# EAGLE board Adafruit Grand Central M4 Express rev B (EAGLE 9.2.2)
REV: B
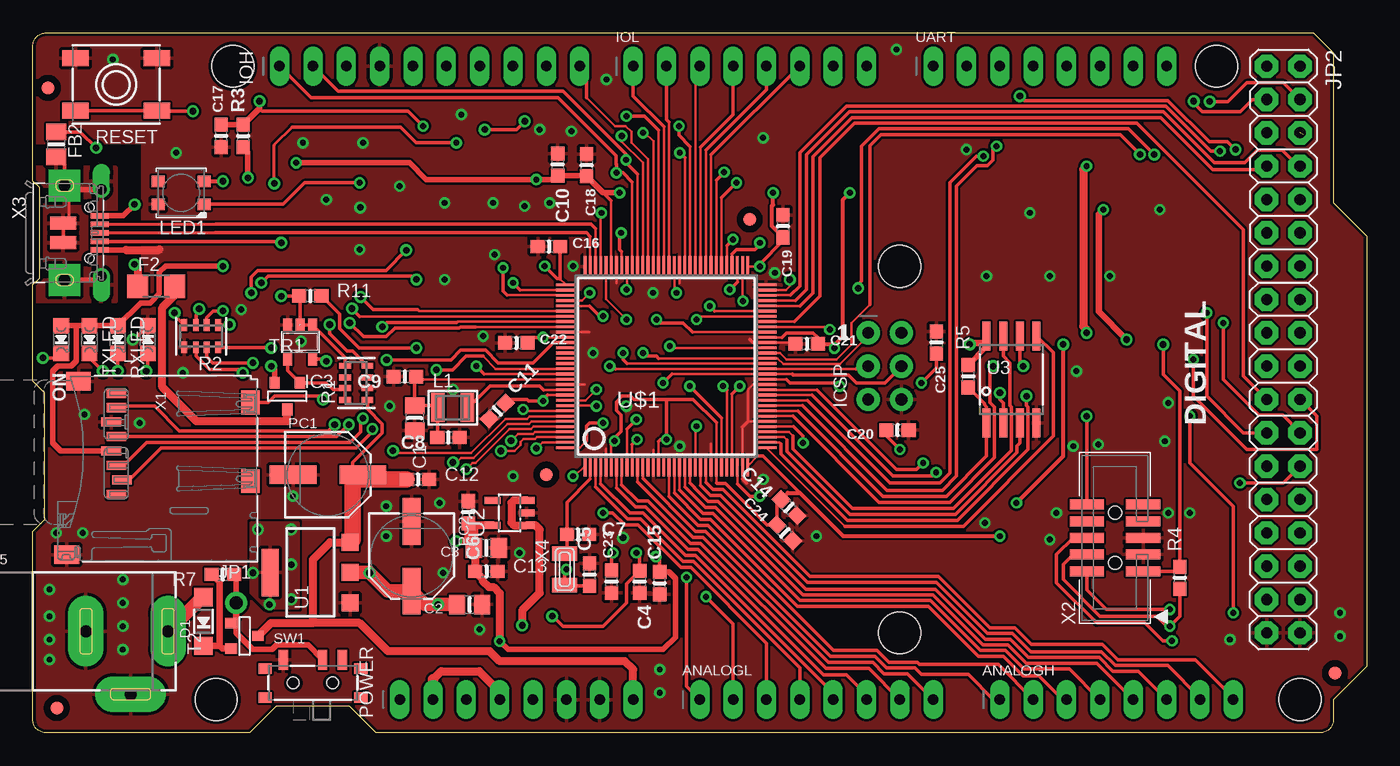
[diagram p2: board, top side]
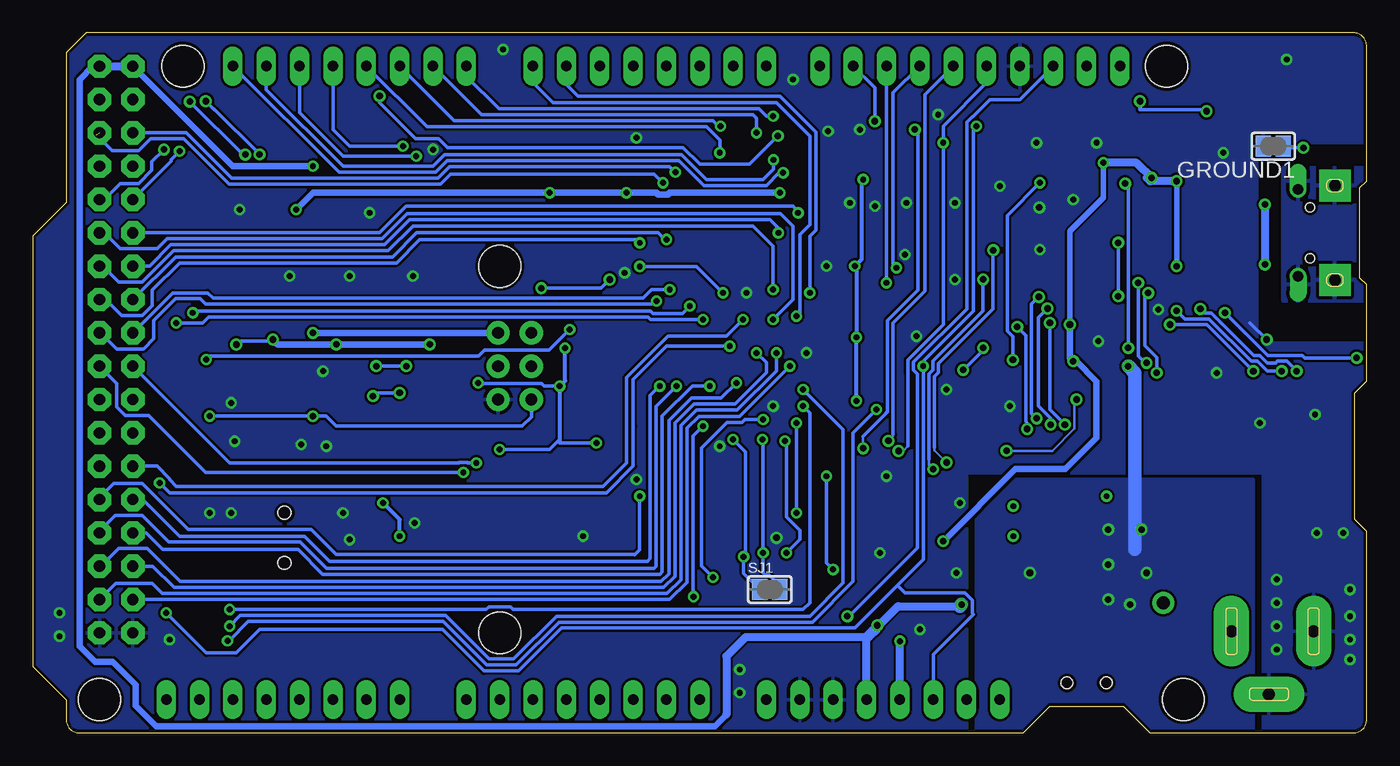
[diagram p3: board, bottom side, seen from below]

Size 101.6 x 53.34 mm. Coordinates in mm from the lower left corner, seen from the top.
Outline: 97.54,53.34 99.06,51.82 99.06,40.39 101.6,37.85 101.6,5.08 99.06,2.54 99.06,1 arc-90 98.06,0 26.16,0 24.13,2.03 18.54,2.03 16.51,0 1,0 arc-90 0,1 0,15.37 0.89,16.26 0.89,25.91 0,26.8 0,34.16 0.51,34.67 0.51,41.53 0,42.04 0,52.34 arc-90 1,53.34 97.54,53.34
Copper layers (1*16): Top 0.035mm / dielectric 1.5mm / Bottom 0.035mm
Design rules "adafruit *": minimum track width 7mil, minimum drill 15.5mil, track to track 7mil, track to pad 7mil, pad to pad 7mil, via to via 7mil, smd to smd 7mil, copper to edge 10mil, drill to drill 8mil, minimum pad ring 10mil, minimum via ring 8mil, stop-mask expansion 2mil, vias tented up to drill 20mil, thermal gap 10mil
Holes 3.2 mm at 66.04,35.56 66.04,7.62 15.24,50.8 13.97,2.54 96.52,2.54 90.17,50.8

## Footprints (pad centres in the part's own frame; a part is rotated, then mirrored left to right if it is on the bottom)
1X08_OVALWAVE = drill 0.8 pad 1.5 long: 1 -8.89,0; 2 -6.35,0; 3 -3.81,0; 4 -1.27,0; 5 1.27,0; 6 3.81,0; 7 6.35,0; 8 8.89,0
0805-NO = smd 1.24 x 1.5: 1 -0.95,0; 2 0.95,0
0603-NO = smd 1.075 x 1: 1 -0.85,0; 2 0.85,0
SOD-123 = smd 1.4 x 1.4: A 1.85,0; C -1.85,0
R1206 = smd 1.6 x 1.803: 1 -1.422,0; 2 1.422,0
FIDUCIAL_1MM = smd 1 x 1: 1 0,0
SOLDERJUMPER_CLOSEDWIRE = smd 1.168 x 1.6: 1 -0.762,0; 2 0.762,0 | smd 0.635 x 0.203: WIRE 0,0
SOT23-5 = smd 0.69 x 0.99: 1 -0.95,-1.29; 2 0,-1.29; 3 0.95,-1.29; 4 0.95,1.3; 5 -0.95,1.3
2X03_ROUND_70MIL = drill 0.9 pad 1.778: 1 -2.54,-1.27; 2 -2.54,1.27; 3 0,-1.27; 4 0,1.27; 5 2.54,-1.27; 6 2.54,1.27
1X10_OVALWAVE = drill 0.8 pad 1.5 long: 1 -11.43,0; 2 -8.89,0; 3 -6.35,0; 4 -3.81,0; 5 -1.27,0; 6 1.27,0; 7 3.81,0; 8 6.35,0; 9 8.89,0; 10 11.43,0
1X01_ROUND = drill 1 pad 1.676: 1 0,0
2X18_THICKWAVE = drill 0.85 pad 1.778 octagon: 1 -21.59,-1.27; 2 -21.59,1.27; 3 -19.05,-1.27; 4 -19.05,1.27; 5 -16.51,-1.27; 6 -16.51,1.27; 7 -13.97,-1.27; 8 -13.97,1.27; 9 -11.43,-1.27; 10 -11.43,1.27; 11 -8.89,-1.27; 12 -8.89,1.27; 13 -6.35,-1.27; 14 -6.35,1.27; 15 -3.81,-1.27; 16 -3.81,1.27; 17 -1.27,-1.27; 18 -1.27,1.27; 19 1.27,-1.27; 20 1.27,1.27; 21 3.81,-1.27; 22 3.81,1.27; 23 6.35,-1.27; 24 6.35,1.27; 25 8.89,-1.27; 26 8.89,1.27; 27 11.43,-1.27; 28 11.43,1.27; 29 13.97,-1.27; 30 13.97,1.27; 31 16.51,-1.27; 32 16.51,1.27; 33 19.05,-1.27; 34 19.05,1.27; 35 21.59,-1.27; 36 21.59,1.27
CHIPLED_0805_NOOUTLINE = smd 1.2 x 1.2: A 0,-1.05; C 0,1.05
INDUCTOR_1007 = smd 1.016 x 2.2: P$1 -1.127,0; P$2 1.127,0
LED3535 = smd 1 x 0.85: 1 -1.75,0.875; 2 -1.75,-0.875; 3 1.75,-0.875; 4 1.75,0.875
PANASONIC_D = smd 3.556 x 1.4: + 2.654,0; - -2.654,0
RESPACK_4X0603 = smd 0.45 x 0.9: 1 -1.3,-0.85; 2 -0.4,-0.85; 3 0.4,-0.85; 4 1.3,-0.85; 5 1.3,0.85; 6 0.4,0.85; 7 -0.4,0.85; 8 -1.3,0.85
EVQ-Q2_SMALLER = smd 2 x 1.2: A -3.1,-2; A' 3.1,-2; B -3.1,2; B' 3.1,2
SPDT_SMT_SSSS811101 = smd 0.7 x 1.5: A -2.25,1.75; B 0.75,1.75; C 2.25,1.75 | smd 1 x 0.8: SUP1 -3.65,1.1; SUP2 -3.65,-1.1; SUP3 3.65,1.1; SUP4 3.65,-1.1 | hole 0.9: -1.5,0; 1.5,0
SOT-23 = smd 0.787 x 0.889: 1 0.025,-1.016; 2 -0.94,1.016; 3 0.991,1.016
SOT223-R = smd 1.3 x 1.3: 1 -2.3,-3.05; 2 0,-3.05; 3 2.3,-3.05 | smd 3.6 x 1.3: 4 0,3.05
SOT23-DBV = smd 0.55 x 1.2: 1 -0.95,-1.3; 2 0,-1.3; 3 0.95,-1.3; 4 0.95,1.3; 5 -0.95,1.3
SOIC8_208MIL = smd 0.6 x 2.2: 1 -1.905,-3.315; 2 -0.635,-3.315; 3 0.635,-3.315; 4 1.905,-3.315; 5 1.905,3.315; 6 0.635,3.315; 7 -0.635,3.315; 8 -1.905,3.315
SQFP-S-14X14-128 = smd 0.2 x 1.6: 1 -6.2,-7.6; 2 -5.8,-7.6; 3 -5.4,-7.6; 4 -5,-7.6; 5 -4.6,-7.6; 6 -4.2,-7.6; 7 -3.8,-7.6; 8 -3.4,-7.6; 9 -3,-7.6; 10 -2.6,-7.6; 11 -2.2,-7.6; 12 -1.8,-7.6; 13 -1.4,-7.6; 14 -1,-7.6; 15 -0.6,-7.6; 16 -0.2,-7.6; 17 0.2,-7.6; 18 0.6,-7.6; 19 1,-7.6; 20 1.4,-7.6; 21 1.8,-7.6; 22 2.2,-7.6; 23 2.6,-7.6; 24 3,-7.6; 25 3.4,-7.6; 26 3.8,-7.6; 27 4.2,-7.6; 28 4.6,-7.6; 29 5,-7.6; 30 5.4,-7.6; 31 5.8,-7.6; 32 6.2,-7.6; 65 6.2,7.6; 66 5.8,7.6; 67 5.4,7.6; 68 5,7.6; 69 4.6,7.6; 70 4.2,7.6; 71 3.8,7.6; 72 3.4,7.6; 73 3,7.6; 74 2.6,7.6; 75 2.2,7.6; 76 1.8,7.6; 77 1.4,7.6; 78 1,7.6; 79 0.6,7.6; 80 0.2,7.6; 81 -0.2,7.6; 82 -0.6,7.6; 83 -1,7.6; 84 -1.4,7.6; 85 -1.8,7.6; 86 -2.2,7.6; 87 -2.6,7.6; 88 -3,7.6; 89 -3.4,7.6; 90 -3.8,7.6; 91 -4.2,7.6; 92 -4.6,7.6; 93 -5,7.6; 94 -5.4,7.6; 95 -5.8,7.6; 96 -6.2,7.6 | smd 1.6 x 0.2: 33 7.6,-6.2; 34 7.6,-5.8; 35 7.6,-5.4; 36 7.6,-5; 37 7.6,-4.6; 38 7.6,-4.2; 39 7.6,-3.8; 40 7.6,-3.4; 41 7.6,-3; 42 7.6,-2.6; 43 7.6,-2.2; 44 7.6,-1.8; 45 7.6,-1.4; 46 7.6,-1; 47 7.6,-0.6; 48 7.6,-0.2; 49 7.6,0.2; 50 7.6,0.6; 51 7.6,1; 52 7.6,1.4; 53 7.6,1.8; 54 7.6,2.2; 55 7.6,2.6; 56 7.6,3; 57 7.6,3.4; 58 7.6,3.8; 59 7.6,4.2; 60 7.6,4.6; 61 7.6,5; 62 7.6,5.4; 63 7.6,5.8; 64 7.6,6.2; 97 -7.6,6.2; 98 -7.6,5.8; 99 -7.6,5.4; 100 -7.6,5; 101 -7.6,4.6; 102 -7.6,4.2; 103 -7.6,3.8; 104 -7.6,3.4; 105 -7.6,3; 106 -7.6,2.6; 107 -7.6,2.2; 108 -7.6,1.8; 109 -7.6,1.4; 110 -7.6,1; 111 -7.6,0.6; 112 -7.6,0.2; 113 -7.6,-0.2; 114 -7.6,-0.6; 115 -7.6,-1; 116 -7.6,-1.4; 117 -7.6,-1.8; 118 -7.6,-2.2; 119 -7.6,-2.6; 120 -7.6,-3; 121 -7.6,-3.4; 122 -7.6,-3.8; 123 -7.6,-4.2; 124 -7.6,-4.6; 125 -7.6,-5; 126 -7.6,-5.4; 127 -7.6,-5.8; 128 -7.6,-6.2
MICROSD = smd 0.7 x 1.5: 1 9,-10.64; 2 7.9,-10.24; 3 6.8,-10.64; 4 5.7,-11.04; 5 4.6,-10.64; 6 3.5,-11.04; 7 2.4,-10.64; 8 1.3,-10.64 | smd 1.8 x 1.4: CD1 2,-0.44; CD2 8,-0.44 | smd 1.4 x 1.9: MT1 0.4,-13.54; MT2 13.6,-14.44
2X05_1.27MM_BOX_POSTS = smd 0.76 x 2.6: 1 -2.54,-2.15; 2 -2.54,2.15; 3 -1.27,-2.15; 4 -1.27,2.15; 5 0,-2.15; 6 0,2.15; 7 1.27,-2.15; 8 1.27,2.15; 9 2.54,-2.15; 10 2.54,2.15 | hole 1: -1.905,0; 1.905,0
4UCONN_20329_V2 = smd 1 x 2: BASE@1 -0.75,-2; BASE@2 0.75,-2 | smd 0.4 x 1.35: D+ 0,0.775; D- -0.65,0.775; GND 1.3,0.775; ID 0.65,0.775; VBUS -1.3,0.775 | drill 0.8 pad 1.143 offset: SPRT@1 -3.3,0.9; SPRT@2 3.3,0.9 | drill 0.9 pad 2.413 square: SPRT@3 -3.6,-1.9; SPRT@4 3.6,-1.9 | hole 0.7: -1.95,0; 1.95,0
XTAL3215 = smd 1.1 x 1.9: P$1 1.2,0; P$2 -1.2,0
DCJACK_2MM_PTH = drill 0.9 pad 2.7 long: GND 7.35,0; GNDBREAK 10.75,-4.8; PWR 13.6,0

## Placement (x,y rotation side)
ANALOGH  20610  [1X08_OVALWAVE]  82.55,2.54 0 top
ANALOGL  20610  [1X08_OVALWAVE]  59.69,2.54 0 top
C1  10uF  [0805-NO]  29.09,23.98 270 top
C2  10uF  [0805-NO]  33.27,9.78 180 top
C3  10uF  [0805-NO]  34.54,14.1 180 top
C4  .1u  [0603-NO]  46.23,11.51 270 top
C5  22pF  [0603-NO]  42.42,12.06 90 top
C6  .1u  [0603-NO]  33.17,16.8 270 top
C7  22pF  [0603-NO]  41.53,15.11 0 top
C8  .1u  [0603-NO]  31.67,22.5 180 top
C9  1uF  [0603-NO]  28.34,27.14 180 top
C10  .1u  [0603-NO]  39.98,43.3 270 top
C11  .1u  [0603-NO]  35.38,24.53 45 top
C12  0.1uF  [0603-NO]  29.34,19.3 0 top
C13  0.1uF  [0603-NO]  34.54,12.32 0 top
C14  .1u  [0603-NO]  57.6,17.17 135 top
C15  .1u  [0603-NO]  47.75,11.4 90 top
C16  .1u  [0603-NO]  39.32,37.06 0 top
C17  0.1uF  [0603-NO]  14.35,45.49 90 top
C18  .1u  [0603-NO]  42.19,43.26 270 top
C19  .1u  [0603-NO]  57.15,38.61 270 top
C20  .1u  [0603-NO]  65.86,23.06 180 top
C21  .1u  [0603-NO]  58.95,29.64 0 top
C22  .1u  [0603-NO]  36.83,29.72 0 top
C23  .1u  [0603-NO]  44.07,11.53 90 top
C24  .1u  [0603-NO]  57.28,15.24 135 top
C25  .1u  [0603-NO]  68.83,29.74 270 top
D1  MBR120  [SOD-123]  13,8.48 90 top
F2  500mA  [R1206]  9.4,34.04 0 top
FB2  FERRITE  [0805-NO]  1.78,44.83 270 top
FD1  FIDUCIAL_1MM  [FIDUCIAL_1MM]  1.14,49.15 0 top
FD2  FIDUCIAL_1MM  [FIDUCIAL_1MM]  99.18,4.55 0 top
FD3  FIDUCIAL_1MM  [FIDUCIAL_1MM]  1.82,1.89 0 top
FD4  FIDUCIAL_1MM  [FIDUCIAL_1MM]  39.12,19.68 0 top
FD5  FIDUCIAL_1MM  [FIDUCIAL_1MM]  54.61,39.12 0 top
GROUND1  [SOLDERJUMPER_CLOSEDWIRE]  7.11,44.7 180 bottom
IC3  74LVC1G125D  [SOT23-5]  20.37,29.79 180 top
ICSP  3x2 M  [2X03_ROUND_70MIL]  64.9,27.94 270 top
IOH  20611  [1X10_OVALWAVE]  30.23,50.8 0 top
IOL  20610  [1X08_OVALWAVE]  54.61,50.8 0 top
JP1  [1X01_ROUND]  15.49,9.91 0 top
JP2  [2X18_THICKWAVE]  95.25,29.21 270 top
L  RED  [CHIPLED_0805_NOOUTLINE]  8.76,29.97 0 top
L1  10uH  [INDUCTOR_1007]  31.98,24.79 0 top
LED1  WS2812B3535  [LED3535]  11.3,41.15 180 top
ON  GREEN  [CHIPLED_0805_NOOUTLINE]  2.16,29.97 180 top
PC1  47uF/25V  [PANASONIC_D]  22.48,19.66 0 top
PC2  47uF+/6.3V+  [PANASONIC_D]  28.85,13.46 270 top
POWER  20610  [1X08_OVALWAVE]  36.83,2.54 0 top
R1  100K  [RESPACK_4X0603]  24.64,26.67 90 top
R2  1K  [RESPACK_4X0603]  12.83,30.23 180 top
R3  10K  [0603-NO]  16.02,45.48 90 top
R4  1K  [0603-NO]  87.38,11.81 90 top
R5  10K  [0603-NO]  71.25,27.18 90 top
R7  10K  [0603-NO]  14.48,12.06 180 top
R11  330R  [0603-NO]  21.13,33.3 0 top
RESET  EVQQ 6mm  [EVQ-Q2_SMALLER]  6.35,49.4 180 top
RXLED  YELLOW  [CHIPLED_0805_NOOUTLINE]  6.48,29.97 180 top
SJ1  AREF_3V  [SOLDERJUMPER_CLOSEDWIRE]  45.47,10.92 0 bottom
SW1  [SPDT_SMT_SSSS811101]  21.34,3.81 0 top
T2  DMP3098L-7  [SOT-23]  16.13,7.37 90 top
TR1  DMP3098L-7  [SOT-23]  19.35,25.65 0 top
TXLED  YELLOW  [CHIPLED_0805_NOOUTLINE]  4.32,29.97 180 top
U1  NCP1117ST50T3G  [SOT223-R]  21.13,12.22 90 top
U2  AP2112K-3.3  [SOT23-DBV]  36.32,16.76 90 top
U3  GD25Q64  [SOIC8_208MIL]  74.55,26.92 0 top
U$1  SAMD51PXXA  [SQFP-S-14X14-128]  48.26,27.94 0 top
U$23  [GRANDCENTRAL_REVB-BOT]  101.6,0 0 bottom
U$30  [GRANDCENTRAL_REVB_TOP]  0,0 0 top
UART  20610  [1X08_OVALWAVE]  77.47,50.8 0 top
X1  microsd  [MICROSD]  17.02,27.18 270 top
X2  2x5 0.05" SWD  [2X05_1.27MM_BOX_POSTS]  82.42,14.86 90 top
X3  20329  [4UCONN_20329_V2]  4.32,38.1 270 top
X4  32.768  [XTAL3215]  40.51,12.45 270 top
X5  2.1mm  [DCJACK_2MM_PTH]  -3.3,7.75 0 top

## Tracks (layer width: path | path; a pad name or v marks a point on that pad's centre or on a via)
3.3V  (via drill 0.45, 0.5)
  Top 0.178: 52.06,19.06 U$1.26 52.06,23.63 | U$1.15 47.66,22.19 | U$1.6 44.06,21.99 | U$1.46 57.39,26.94 | U$1.37 57.94,23.34 | U$1.65 v55.37,35.54 | U$1.107 v38.86,30.14 | U$1.91 44.06,40.54 | U$1.54 57.06,30.14 | U$1.79 48.86,33.69 | U$1.118 39.2,25.74 | U$1.32 55.2,21.08
  Top 0.203: U$1.97 40.6,34.14 40.17,34.58
  Top 0.254: 52.06,19.06 52.12,19 52.77,19 55.93,15.84 C24.2 56.68,17.45 C14.2 | C15.2 47.75,13.13 v47.46,13.42 | C23.2 44.07,13.59 v44.2,13.72 | 44.06,21.99 v44.31,22.24 44.31,22.47 44.79,22.95 44.79,24.24 44.45,24.58 44.45,25.21 44.9,25.65 44.95,25.65 44.96,25.65 45.53,25.65 45.78,25.4 48.26,25.4 | 57.39,26.94 57.66,26.67 61.21,26.67 v61.47,26.42 | 57.94,23.34 58.67,22.61 v58.67,22.1 | v38.86,30.14 38.1,30.14 C22.2 | 44.06,40.54 43.44,41.16 42.3,42.3 C18.2 | 57.06,30.14 57.4,30.48 59.44,30.48 59.8,30.11 C21.2 | 48.86,33.69 v49.02,33.53 | v38.99,35.56 39.94,34.61 40.17,34.61 | 39.2,25.74 38.86,25.4 v38.86,25.3 37.75,25.3 37.65,25.4 36.25,25.4 C11.2 | 52.06,23.63 50.29,25.4 48.26,25.4 | 47.66,22.19 47.82,22.35 v48.26,22.35 48.26,25.4 | 55.2,21.08 55.63,21.08 58.42,18.29 | 40.17,34.58 40.17,34.61 | 40.17,34.61 C16.2 | v55.37,35.54 55.37,35.73 57.15,37.5 C19.2 | X2.1 87.03,12.32 R4.2 87.38,26.04 86.11,27.3 v86.11,29.59 | R1.4 24.38,29.08 23.93,29.08 22.61,30.41 v22.61,31.11 | v22.35,28.32 22.18,28.49 IC3.5 | C20.2 65.01,22.62 v66.04,21.59 | v67.69,26.67 68.83,27.81 C25.2
  Top 0.305: LED1.2 13.07,42.04 v14.48,42.04 | v56.39,41.15 56.39,40.24 56.29,40.14 56.29,38.61 C19.2 | C21.2 60.96,29.64 | 60.96,29.64 61.14,29.64 61.72,30.23 61.72,40.64 v62.23,41.15 | v61.06,29.31 60.96,29.41 60.96,29.64 | C14.2 57.51,18.29 58.42,18.29 61.72,14.99 v73.66,14.99 | v78.49,29.59 78.49,21.08 v74.93,17.53
  Top 0.406: R3.1 16.38,44.27 v16.38,42.29 | v20.07,43.43 28.7,43.43 29.97,42.16 v38.35,42.16 39.7,42.16 C10.2 42.15,42.45 42.3,42.3 | C18.2 43.44,41.16 v44.7,41.16 v44.7,41.15 | C15.2 48.45,12.26 48.95,11.76 48.95,7.29 48.01,6.35 36.2,6.35 v35.56,6.99 | ON.A 3.3,31.02 | 3.3,31.02 TXLED.A RXLED.A 8.21,32.75 8.93,32.75 9.64,33.46 9.64,35.09 10.1,35.56 v14.48,35.56 | R5.2 72.64,29.43 72.64,29.72 U3.8 | X1.4 2.14,21.48 1.52,22.1 1.52,27.56 1.91,27.94 2.92,27.94 3.3,28.33 3.3,31.02
  Top 0.508: v71.37,29.59 71.5,29.72 72.64,29.72 | v83.31,29.97 81.18,32.1 81.18,39.53 v81.53,39.88
  Top 0.61: U2.5 33.31,15.81 | v35.56,6.99 35.56,10.64 35.09,11.11 34.74,11.11 34.27,11.58 34.27,11.74 C13.1 33.69,14 C3.2 33.59,15.53 C6.2 33.17,14.61 v32.26,14.61 | 30.48,4.06 31.11,4.7 34.01,4.7 35.56,3.15 POWER.4
  Top 0.813: 30.48,4.06 POWER.2
  Top 1.016: 33.31,15.81 C6.2
  Bottom 0.254: v61.47,26.42 62.66,26.42 62.87,26.62 67.64,26.62 v67.69,26.67 | 61.47,22.1 v58.67,22.1 | v49.02,33.53 51.03,35.54 v55.37,35.54 | v44.2,13.72 43.18,14.73 43.18,15.44 44.19,16.45 44.19,22.12 v44.31,22.24 | v48.26,22.35 47.33,21.42 47.33,13.55 v47.46,13.42 47.46,12.15 SJ1.1 | 61.47,22.35 62.23,21.59 v66.04,21.59 | v86.11,29.59 85.98,29.59 85.72,29.85 83.19,29.85
  Bottom 0.305: 16.76,42.29 v16.38,42.29 | v61.06,29.31 61.06,26.82 v61.47,26.42 61.47,22.35 61.47,22.1 | v38.35,42.16 38.48,42.04 38.48,36.07 v38.99,35.56 38.86,35.43 v38.86,30.14 v38.86,25.3 | v73.66,14.99 73.66,16.26 v74.93,17.53
  Bottom 0.406: v14.48,35.56 14.48,41.78 14.73,42.04 | v22.61,31.11 22.61,38.23 20.07,40.77 v20.07,43.43
  Bottom 0.508: v81.53,39.88 80.26,41.15 v62.23,41.15 v56.39,41.15 54.08,41.15 53.96,41.02 53.23,41.02 53.1,41.15 v44.7,41.15 | v71.37,29.59 v78.49,29.59 82.94,29.59 83.19,29.85 | v32.26,14.61 26.76,20.11 22.93,20.11 20.58,22.46 20.58,26.78 22.12,28.32 v22.35,28.32 22.61,28.57 v22.61,31.11
  Bottom 0.61: v14.48,42.04 14.73,42.04 16.51,42.04 16.76,42.29 | v16.38,42.29 17.53,43.43 v20.07,43.43 | POWER.4 v35.56,6.99
!RESET  (via drill 0.45, 0.5)
  Top 0.178: U$1.114 34.38,27.34
  Top 0.254: RESET.B' RESET.B 9.78,47.37 v12.19,47.37 | 34.38,27.34 v33.78,27.94 | v29.72,46.23 28.57,47.37 17.49,47.37 17.27,47.59 | v88.14,24.13 88.14,20.57 91.44,17.27 v91.44,9.14 | X2.10 80.27,24.12 v80.26,24.13
  Top 0.406: v17.27,48.13 17.27,47.59 R3.2 14.36,46.33 C17.2
  Bottom 0.254: v12.19,47.37 12.32,47.5 17.27,47.5 | v88.14,24.13 v80.26,24.13 79.25,24.13 78.49,23.37 64.33,23.37 63.63,24.07 ICSP.5 | v29.72,46.23 29.97,45.97 29.97,32.13 33.78,28.32 v33.78,27.94 33.78,13.21 35.75,11.24 | 35.75,11.24 38.99,8 61.32,8 64.59,4.72 67.24,4.72 70.39,7.87 84.33,7.87 86.11,6.1 88.39,6.1 v91.44,9.14 | POWER.3 33.02,5.97 29.97,9.02 30.05,9.09 30.05,10.12 30.6,10.67 35.18,10.67 35.75,11.24
  Bottom 0.305: v17.27,48.13 17.27,47.5
+5V  (via drill 0.45, 0.5)
  Top 0.406: TR1.2 18.41,27.69 v18.16,27.94
  Top 0.61: U2.3 36.64,17.71 36.45,17.53 36.45,16 36.64,15.81 U2.1 38.29,15.81 38.61,15.49 38.61,10.67 37.27,9.34 v37.27,8.19 | v80.26,43.18 80.01,42.93 80.01,30.99 80.26,30.73 v80.26,30.48
  Top 1.016: U1.2 25.63,12.22 v25.65,12.19 27.04,10.81 PC2.+ 29.88,9.78 v30.86,9.78 C2.2
  Bottom 0.508: JP2.1 86.36,43.18 v80.26,43.18 | JP2.2 97.03,50.8 98.04,49.78 98.04,6.6 96.85,5.41 95.52,5.41 93.78,3.67 93.78,2.08 92.2,0.51 49.65,0.51 48.77,1.39 | v80.26,30.48 ICSP.2
  Bottom 0.61: JP2.2 JP2.1 | POWER.5 38.1,7.37 v37.27,8.19 | v37.27,8.19 37.15,8.19 35.69,9.65 30.99,9.65 | 48.77,1.39 48.77,5.84 47.3,7.32 37.9,7.32 37.27,7.94 v37.27,8.19
  Bottom 1.016: 30.99,9.65 v30.86,9.78 | 17.65,13.97 17.65,27.43 v18.16,27.94
  other vias: 19.68,12.83 19.68,15.49 19.68,10.16 16.76,12.19 18.03,9.78 17.14,15.49
  pour Bottom: 8.64,19.3 29.72,19.3 29.72,0.25 8.64,0.25
  pour Top: 16.64,16 16.64,10.67 17.78,9.53 20.19,9.53 20.19,15.75 20.19,16
A0  (via drill 0.45)
  Top 0.178: U$1.9 45.26,23.16
  Top 0.254: v49.78,11.84 49.78,3.56 ANALOGL.1 | 45.26,23.16 v45.97,23.88
  Bottom 0.254: v49.78,11.84 50.67,12.73 50.67,21.72 48.72,23.67 47.57,23.67 47.36,23.88 v45.97,23.88
A1  (via drill 0.45)
  Top 0.178: U$1.22 50.46,23.28
  Top 0.254: 50.46,23.28 v50.55,23.37 | v51.27,10.37 53.34,8.3 ANALOGL.2
  Bottom 0.254: v50.55,23.37 51.31,22.61 51.31,10.41 v51.27,10.37
A2  (via drill 0.45)
  Top 0.178: U$1.128 41.68,21.74
  Top 0.203: 42.16,22.23 41.68,21.74
  Top 0.254: ANALOGL.3 55.88,6.83 50.12,12.6 49.35,12.6 46.12,15.84 45.1,15.84 44.17,16.76 v43.43,16.76 | 42.16,22.23 42.16,23.37 42.42,23.62 v43.43,23.62
  Bottom 0.254: v43.43,16.76 v43.43,23.62
A3
  Top 0.178: U$1.3 42.86,18.72
  Top 0.254: ANALOGL.4 58.42,4.94 50.3,13.06 49.54,13.06 46.31,16.29 45.29,16.29 42.86,18.72
A4
  Top 0.178: U$1.4 43.26,18.97
  Top 0.254: ANALOGL.5 60.96,3.05 50.49,13.51 49.73,13.51 46.5,16.75 45.48,16.75 43.26,18.97
A5
  Top 0.178: U$1.7 44.46,18.65
  Top 0.254: ANALOGL.6 63.5,2.89 61.96,4.43 60.23,4.43 50.68,13.97 49.92,13.97 46.69,17.21 45.9,17.21 44.46,18.65
A6
  Top 0.178: U$1.8 44.86,18.89
  Top 0.254: ANALOGL.7 63.68,4.9 60.4,4.9 50.87,14.43 50.11,14.43 46.87,17.66 46.09,17.66 44.86,18.89
A7
  Top 0.178: U$1.11 46.06,19.12
  Top 0.254: ANALOGL.8 66.62,4.5 64.84,4.5 63.98,5.36 60.59,5.36 51.06,14.88 50.3,14.88 46.06,19.12
A8
  Top 0.178: U$1.12 46.46,19.37
  Top 0.254: 46.46,19.37 50.49,15.34 51.25,15.34 60.75,5.84 64.14,5.84 65.02,4.95 67.18,4.95 67.69,4.45 71.25,4.45 73.15,2.54 ANALOGH.1
A9
  Top 0.178: U$1.17 48.46,18.02
  Top 0.254: 48.46,18.02 50.68,15.8 51.44,15.8 60.97,6.27 64.31,6.27 65.2,5.38 67.36,5.38 67.54,5.21 73.53,5.21 ANALOGH.2
A10
  Top 0.178: U$1.18 48.86,18.27
  Top 0.254: 48.86,18.27 50.87,16.26 51.63,16.26 58.23,9.65 68.2,9.65 72.01,5.84 73.91,5.84 75.41,4.34 76.64,4.34 78.44,2.54 ANALOGH.3
A11
  Top 0.178: U$1.19 49.26,18.51
  Top 0.254: 49.26,18.51 51.06,16.71 51.82,16.71 58.45,10.08 68.38,10.08 72.19,6.27 74.09,6.27 75.49,4.88 78.94,4.88 ANALOGH.4
A12
  Top 0.178: U$1.20 49.66,18.76
  Top 0.254: 49.66,18.76 51.25,17.17 52.01,17.17 58.66,10.52 68.56,10.52 72.37,6.71 74.27,6.71 75.67,5.31 81.05,5.31 ANALOGH.5
A13
  Top 0.178: U$1.21 50.06,19.03
  Top 0.254: 50.06,19.03 50.4,18.68 50.4,18.66 51.44,17.63 52.2,17.63 58.88,10.95 68.74,10.95 72.55,7.14 74.45,7.14 75.85,5.74 81.23,5.74 82.27,4.7 84.2,4.7 ANALOGH.6
A14
  Top 0.178: U$1.23 50.86,18.85
  Top 0.254: 50.86,18.85 51.63,18.09 52.39,18.09 58.99,11.48 68.81,11.48 72.72,7.57 74.63,7.57 76.03,6.17 81.41,6.17 82.45,5.13 86.44,5.13 88.9,2.67 ANALOGH.7
A15
  Top 0.178: U$1.24 51.26,19.1
  Top 0.254: 51.26,19.1 51.82,18.54 52.58,18.54 59.21,11.91 68.99,11.91 72.9,8 74.81,8 76.08,6.73 81.46,6.73 82.63,5.56 88.54,5.56 91.44,2.67 ANALOGH.8
AREF  (via drill 0.45, 0.5)
  Top 0.178: U$1.10 45.66,21.99
  Top 0.254: v45.97,13.72 46.23,13.46 C4.1 45.21,11.34 45.21,9.91 43.43,8.13 40.39,8.13 39.63,8.89 v39.56,8.89 | 45.66,21.99 v46.02,22.35
  Bottom 0.254: v46.02,22.35 45.97,22.31 v45.97,13.72 45.97,12.19 45.81,12.03 45.52,12.03 44.84,11.35 44.84,11.06 SJ1.2 | v39.56,8.89 39.43,8.89 34.21,14.1 34.21,27.34 34.52,27.64 34.52,28.24 30.45,32.31 30.45,46.53 30.02,46.96 30,46.96 28.7,48.26 26.42,48.26 IOH.3
D0  (via drill 0.45)
  Top 0.178: U$1.101 42.39,32.54
  Top 0.254: 42.39,32.54 43.18,31.75 v43.43,31.75
  Bottom 0.254: IOL.8 63.5,49.53 61.98,48.01 44.96,48.01 42.42,45.47 42.42,38.73 43.18,37.98 43.18,32.01 v43.43,31.75
D1  (via drill 0.45)
  Top 0.178: U$1.100 41.83,32.94 v42.42,33.53
  Bottom 0.254: IOL.7 60.96,49.4 60.07,48.51 44.7,48.51 41.96,45.77 41.96,38.3 42.42,37.85 v42.42,33.53
D2
  Top 0.178: U$1.72 51.66,44.04
  Top 0.254: 51.66,44.04 IOL.6
D3
  Top 0.178: U$1.73 51.26,44.4
  Top 0.254: 51.26,44.4 55.88,49.02 IOL.5
D4
  Top 0.178: U$1.74 50.86,44.64
  Top 0.254: IOL.4 53.34,47.12 50.86,44.64
D5
  Top 0.178: U$1.75 50.46,50.46
  Top 0.254: 50.46,50.46 IOL.3
D6
  Top 0.178: U$1.80 48.46,46.54
  Top 0.254: 48.46,46.54 48.26,46.74 IOL.2
D7
  Top 0.178: U$1.81 48.06,46.17
  Top 0.254: 48.06,46.17 45.72,48.51 IOL.1
D8
  Top 0.178: U$1.84 46.86,43.7
  Top 0.203: 46.86,43.7 45.59,44.98 45.59,45.79 45.16,46.22 44.34,46.22 42.16,48.4
  Top 0.254: IOH.10 42.16,50.29 42.16,48.4
D9  (via drill 0.5)
  Top 0.203: U$1.127 38.82,22.14 v38.35,21.67
  Top 0.254: v34.42,45.97 36.83,45.97 v37.47,46.61
  Bottom 0.203: v38.35,21.67 v38.36,21.68 38.36,22.6
  Bottom 0.254: 38.36,22.6 37.05,23.91 37.03,23.91 36.6,24.33 36.6,24.36 36.5,24.46 36.5,31.42 34.16,33.76 34.16,45.85 34.29,45.85 v34.42,45.97 | v37.47,46.61 37.47,49.15 IOH.9
D10  (via drill 0.45)
  Top 0.178: U$1.98 37.13,33.74
  Top 0.254: 37.13,33.74 v36.58,34.29
  Bottom 0.254: IOH.8 v36.58,34.29
D11  (via drill 0.45)
  Top 0.178: U$1.99 36.13,33.34
  Top 0.254: 36.13,33.34 35.81,33.66 v35.81,35.43
  Bottom 0.254: IOH.7 36.07,48.77 36.07,35.69 v35.81,35.43
D12  (via drill 0.5)
  Top 0.203: U$1.125 38.26,22.94 38.1,22.79 36.97,22.79 v36.43,22.25
  Bottom 0.203: v36.43,22.25 36.07,22.61 36.07,22.73
  Bottom 0.254: 36.07,22.73 36.07,31.24 33.66,33.65 33.66,48.64 IOH.6
D13  (via drill 0.45, 0.5)
  Top 0.203: U$1.126 38.4,22.54 38.26,22.41 37.39,22.41 37.16,22.17 37.16,21.94 36.7,21.48 v35.66,21.48
  Top 0.229: v18.39,41.86 18.39,44.81 19.74,46.15
  Top 0.254: 19.74,46.15 28.02,46.15 29.21,44.96 v32.26,44.96 | R2.8 18.12,29.38 v18.16,29.34
  Bottom 0.203: v35.66,21.48 35.29,21.48 34.92,21.84
  Bottom 0.254: IOH.5 28.96,49.53 32.26,46.23 v32.26,44.96 32.26,31.11 34.95,28.42 34.95,27.46 34.92,27.44 34.92,21.84 | v18.16,29.34 18.16,41.63 v18.39,41.86
D22  (via drill 0.5)
  Top 0.178: U$1.51 56.91,28.94 57.4,28.45 61.22,28.45 62.36,29.59 62.36,31.24 63.75,32.64
  Top 0.254: 63.75,32.64 63.75,44.73 64.62,45.59 82.82,45.59 v84.33,44.08 | v88.43,48.13 88.43,47.99 89.07,47.35 91.98,47.35 92.89,48.26 JP2.3
  Bottom 0.254: v84.33,44.08 87.77,47.51 87.77,47.48 v88.43,48.13
D23  (via drill 0.5)
  Top 0.178: U$1.63 57.36,33.74 57.91,34.29 v57.66,34.54
  Top 0.254: v62.87,33.88 62.87,34.16 63.12,34.42 63.12,44.7 64.44,46.02 83.46,46.02 v85.42,44.06 | JP2.4 95.25,49.53 92.46,49.53 91.04,48.11 v89.64,48.11
  Bottom 0.254: v57.66,34.54 58.32,33.88 v62.87,33.88 | v85.42,44.06 85.59,44.06 v89.64,48.11
D44  (via drill 0.45)
  Top 0.178: U$1.55 50.23,30.54
  Top 0.254: 50.23,30.54 49.53,31.24 47.75,31.24 v47.5,31.5
  Bottom 0.254: JP2.25 92.14,20.32 91.19,19.36 91.19,19.31 90.68,18.8 58.17,18.8 56.39,20.57 56.39,27.06 53.23,30.22 48.77,30.22 v47.5,31.5
D45  (via drill 0.45)
  Top 0.178: U$1.52 48.64,29.34
  Top 0.254: 48.64,29.34 v48.51,29.46 | v91.95,19.05 95.25,19.05 JP2.26
  Bottom 0.254: v48.51,29.46 53.34,29.46 55.88,26.92 55.88,23.37 55.88,20.32 57.91,18.29 91.19,18.29 v91.95,19.05
D46  (via drill 0.45)
  Top 0.178: U$1.29 53.26,25.83
  Top 0.254: 53.26,25.83 v53.85,26.42
  Bottom 0.254: JP2.27 93.22,17.78 90.42,14.99 80.9,14.99 78.99,13.08 54.77,13.08 54.57,13.28 54.57,25.69 v53.85,26.42
D47  (via drill 0.45)
  Top 0.178: U$1.30 53.66,18.98
  Top 0.254: v55.37,18.03 54.61,18.03 53.66,18.98
  Bottom 0.254: JP2.28 96.52,17.93 95.45,19 93.27,19 89.77,15.49 80.39,15.49 78.49,13.59 55.77,13.59 55.75,13.57 55.37,13.96 v55.37,18.03
D48  (via drill 0.45)
  Top 0.178: U$1.27 52.46,23.99
  Top 0.254: 52.46,23.99 v50.04,26.42
  Bottom 0.254: JP2.29 92.96,15.24 91.69,13.97 81.41,13.97 79.51,12.08 53.83,12.08 53.66,12.25 53.66,24.13 51.37,26.42 v50.04,26.42
D49  (via drill 0.45)
  Top 0.178: U$1.28 52.86,26.13
  Top 0.254: 52.86,26.13 v52.58,26.42
  Bottom 0.254: JP2.30 96.52,15.39 95.32,16.59 93.27,16.59 91.24,14.55 81.22,14.55 79.21,12.53 54.28,12.53 54.11,12.7 54.11,24.88 v52.58,26.42
D+
  Top 0.178: U$1.95 42.46,37.8
  Top 0.229: X3.D+ 13.89,38.1
  Top 0.254: 42.46,37.8 42.16,38.1 13.89,38.1
D-
  Top 0.178: U$1.94 42.86,38.42
  Top 0.229: X3.D- 13.95,38.75
  Top 0.254: 42.86,38.42 42.53,38.75 13.95,38.75
FLASH_CS
  Top 0.178: U$1.40 58.26,24.54
  Top 0.254: 58.26,24.54 64.77,18.03 69.6,18.03 72.64,21.08 U3.1 72.64,24.83 72.47,25.01 72.47,25.11 R5.1
FLASH_IO0
  Top 0.178: U$1.33 61.85,15.75
  Top 0.254: 61.85,15.75 70.87,15.75 77.72,22.61 77.72,28.97 U3.5
FLASH_IO1  (via drill 0.5)
  Top 0.178: U$1.34 56.85,22.14 56.99,22
  Top 0.254: 56.99,22 56.99,21.26 62.04,16.2 70.41,16.2 75.79,21.58 75.79,24.84 75.69,24.93 v75.69,25.65 | v73.66,25.91 73.66,25.4 73.91,25.15 U3.2
  Bottom 0.254: v75.69,25.65 75.44,25.91 v73.66,25.91
FLASH_IO2
  Top 0.178: U$1.35 57.22,22.54 57.45,22.31
  Top 0.254: 57.45,22.31 57.45,21.45 62.23,16.66 70.26,16.66 74.95,21.36 74.95,21.86 75.18,22.1 U3.3
FLASH_IO3
  Top 0.178: U$1.36 57.58,22.94 57.91,22.61
  Top 0.254: 57.91,22.61 57.91,21.63 62.42,17.12 70.1,17.12 74.52,21.53 74.52,24.84 74.42,24.93 74.42,28.19 73.91,28.7 U3.7
FLASH_SCK  (via drill 0.5)
  Top 0.178: U$1.39 57.9,24.14
  Top 0.254: 57.9,24.14 64.47,17.58 69.85,17.58 73.25,20.98 73.25,24.84 72.9,25.19 72.9,27.69 v73.15,27.94 | v75.44,27.94 75.18,28.2 U3.6
  Bottom 0.254: v73.15,27.94 v75.44,27.94
GND  (via drill 0.45, 0.5)
  Top 0.178: U$1.78 49.28,35.54 49.28,34.29 | U$1.90 44.45,34.29 | U$1.106 42.36,30.54 | U$1.116 42.03,26.54 | U$1.5 43.66,21.62 | U$1.14 47.26,21.57 | 54.06,19.35 U$1.31 54.06,23.33 | U$1.25 51.66,22 | U$1.38 54.47,23.74 | 54.84,29.74 U$1.53 58.01,29.74 | U$1.45 54.86,26.54
  Top 0.203: 54.47,23.74 54.47,26.08 54.53,26.13 54.53,26.21 54.86,26.54
  Top 0.254: 54.06,19.35 54.36,19.05 | 54.47,23.74 54.06,23.33 | 54.84,29.74 54.61,29.97 | 58.01,29.74 C21.1 | L.C 7.71,29.97 v7.62,29.97
  Top 0.406: X3.GND 7.09,36.8
  Top 0.61: 7.09,36.8 9.62,36.8 9.65,36.83
  Bottom 0.254: v7.62,29.97 8.89,31.24
  other vias: 24.94,40.03 72.64,34.8 77.47,34.8 82.04,34.8 75.95,39.62 85.85,39.88 55.63,45.34 71.12,44.45 42.67,28.96 47.24,33.53 45.21,24.89 55.63,19.3 49.28,21.84 59.69,14.99 56.52,35.05 91.19,7.11 38.61,45.97 32.64,47.12 22.35,40.64 25.15,44.96 20.57,44.96 44.96,14.86 99.57,7.37 99.57,9.14 41.15,35.56 39.37,40.39 24.89,36.83 27.94,41.66 10.92,44.2 3.94,24.26 8.13,23.62 34.04,7.87 31.24,12.19 26.92,17.27 26.92,14.99 30.99,17.53 19.81,18.03 37.08,13.72 36.58,19.56 32,26.16 27.18,24.89 34.29,30.23 11.43,27.43 6.1,51.31 1.78,15.24 3.81,15.24 6.86,6.35 6.86,8.13 6.86,9.91 6.86,11.68 1.27,5.59 1.27,7.11 1.27,8.89 1.27,10.92 47.75,4.83 47.75,3.05 43.69,49.78 65.79,52.07 88.14,16.76 20.45,29.84 15.88,32.26 86.49,16.76 77.98,16.76 77.47,14.73 72.52,16 86.23,22.23 81.15,21.97 79.25,21.84 79.5,27.56 86.49,25.15 41.02,45.85 37.47,40.13 31.37,40.39 35.05,40.39 35.18,36.45 31.37,34.54
  pour Bottom: 0,53.34 101.85,53.34 101.85,-0.25 30.48,0 30.48,19.81 7.87,19.81 7.87,0 0.25,0 0,29.72 8.38,29.72 8.38,44.96 0,44.96
  pour Top (rank 2): 0,53.34 101.85,53.34 101.85,-0.25 0,-0.25 0,29.72 8.38,29.72 8.38,44.96 0,44.96
MISO  (via drill 0.45)
  Top 0.178: 47.66,28.54 U$1.50 56.74,28.54 57.18,28.1 61.47,28.1 63.63,30.26 ICSP.1
  Top 0.254: 47.66,28.54 47.5,28.7 46.74,28.7 v46.48,28.96
  Bottom 0.254: JP2.31 92.46,12.7 90.83,11.07 53.54,11.07 52.68,11.94 52.68,23.6 51.24,25.04 48.13,25.04 45.73,27.44 45.73,28.21 v46.48,28.96
MOSI  (via drill 0.45)
  Top 0.178: 57.85,27.34 U$1.47 48.68,27.34
  Top 0.254: 57.85,27.34 57.91,27.28 62.12,27.28 62.74,26.67 64.9,26.67 ICSP.4 | 48.68,27.34 v48.01,26.67
  Bottom 0.254: JP2.32 96.41,12.7 95.07,14.05 92.89,14.05 90.38,11.53 53.73,11.53 53.14,12.13 53.14,23.79 51.43,25.5 49.18,25.5 v48.01,26.67
N$1  (via drill 0.5)
  Top 0.254: R2.1 14.95,31.08 v14.99,31.11 | v8.64,27.56 8.76,27.69 L.A
  Bottom 0.254: v14.99,31.11 12.19,31.11 v8.64,27.56
N$2  (via drill 0.5)
  Top 0.254: FB2.1 3.62,45.78 v4.83,44.58
  Bottom 0.254: v4.83,44.58 6.22,44.58 GROUND1.1
N$3  (via drill 0.5)
  Top 0.254: R2.4 10.79,31.81 v10.79,32.01 | v0.76,28.57 1.81,28.57 ON.C
  Bottom 0.254: v0.76,28.57 4.72,28.57 4.9,28.75 7.53,28.75 v10.79,32.01
N$4
  Top 0.178: U$1.117 38.88,26.14
  Top 0.254: L1.P$2 33.19,24.79 34.81,26.42 38.61,26.42 38.88,26.14
N$5  (via drill 0.5)
  Top 0.254: R2.2 13.23,31.66 13.72,32.16 v14.48,32.16 | v6.48,27.56 RXLED.C
  Bottom 0.254: v14.48,32.16 13.87,31.55 12.01,31.55 8.78,28.32 8.32,28.32 7.56,27.56 v6.48,27.56
N$7  (via drill 0.5)
  Top 0.254: R2.3 12.43,31.84 12.57,31.98 12.57,32.2 v12.67,32.3 | v5.33,27.56 4.32,28.57 TXLED.C
  Bottom 0.254: v12.67,32.3 12.34,31.98 11.83,31.98 8.6,28.75 8.14,28.75 7.59,28.19 6.91,28.19 6.79,28.32 6.09,28.32 v5.33,27.56
N$9  (via drill 0.45)
  Top 0.178: U$1.1 41.28,19.56
  Top 0.254: 41.28,19.56 v41.15,19.56 | v40.64,12.45 40.51,12.32 X4.P$1 40.54,11.21 C5.1
  Bottom 0.254: v41.15,19.56 41.15,12.95 v40.64,12.45
N$10  (via drill 0.5)
  Top 0.254: R1.5 23.79,28.62 IC3.1 IC3.2 20.37,33.21 R11.1 18.94,33.3 v18.92,33.27 | v18.92,37.34 18.81,37.45 X3.ID
  Bottom 0.254: v18.92,37.34 v18.92,33.27
N$11
  Top 0.254: R1.8 R1.7 23.68,26.16 22.86,26.16 22.35,26.67 TR1.3 19.42,27.59 IC3.4
N$12
  Top 0.178: U$1.2 42.46,19.35
  Top 0.254: 42.46,19.35 40.68,17.57 C7.1 40.68,13.81 X4.P$2
N$15
  Top 0.406: 14.22,11.47 R7.2
  Top 0.508: D1.C 14.22,6.63 | 14.22,11.47 14.22,6.63 | 14.22,6.63 14.43,6.43 T2.2
NEOPIX  (via drill 0.45, 0.5)
  Top 0.178: U$1.108 39.65,29.74
  Top 0.254: LED1.1 19.06,40.27 20.7,41.91 v24.89,41.91 | 39.65,29.74 38.1,28.2 35.44,28.2 34.48,29.16 32.57,29.16 31.84,28.42 v26.95,28.42
  Bottom 0.254: v26.95,28.42 26.95,30.2 27.37,30.63 27.37,39.43 v24.89,41.91
PCC_CLK  (via drill 0.45)
  Top 0.178: U$1.62 57.72,33.34
  Top 0.254: 57.72,33.34 58.42,34.04 58.42,44.2 61.98,47.75 86.29,47.75 89.72,44.32 v90.42,44.32
  Bottom 0.254: v90.42,44.32 91.06,43.69 91.06,43.56 JP2.9
PCC_D0  (via drill 0.45)
  Top 0.178: U$1.66 54.06,32.94
  Top 0.254: 54.06,32.94 v54.1,32.9
  Bottom 0.254: JP2.18 96.41,30.48 95.19,29.26 93.15,29.26 92.38,30.03 92.38,31.43 90.74,33.08 88.86,33.08 88.45,32.66 54.34,32.66 v54.1,32.9
PCC_D1  (via drill 0.45)
  Top 0.178: U$1.67 53.66,34.36
  Top 0.254: 53.66,34.36 v53.09,33.78
  Bottom 0.254: JP2.17 90.93,33.53 88.28,33.53 87.88,33.12 55.13,33.12 54.47,33.78 v53.09,33.78
PCC_D2  (via drill 0.45)
  Top 0.178: U$1.68 53.26,36.5
  Top 0.254: 53.26,36.5 53.59,36.83 54.99,36.83 55.44,37.27 v55.37,37.34
  Bottom 0.254: JP2.16 96.03,33.02 94.81,31.8 93.27,31.8 92.51,32.57 92.51,33.73 90.42,35.81 73.91,35.81 72.13,37.59 55.63,37.59 v55.37,37.34
PCC_D3  (via drill 0.45)
  Top 0.178: U$1.69 52.86,37.12
  Top 0.254: 52.86,37.12 v53.34,37.6
  Bottom 0.254: JP2.15 90.73,36.27 74.21,36.27 72.38,38.1 53.98,38.1 53.47,37.6 v53.34,37.6
PCC_D4  (via drill 0.45)
  Top 0.178: U$1.88 45.26,33.83
  Top 0.254: 45.26,33.83 v45.21,33.78
  Bottom 0.254: JP2.14 96.29,35.56 95.07,34.34 93.27,34.34 90.89,36.73 74.52,36.73 72.64,38.61 46.74,38.61 45.21,37.08 v45.21,33.78
PCC_D5  (via drill 0.45)
  Top 0.178: U$1.89 44.86,36.67
  Top 0.254: 44.86,36.67 44.7,36.83 44.7,37.99 v44.82,38.1
  Bottom 0.254: v44.82,38.1 44.82,38.45 45.47,39.1 72.89,39.1 74.81,37.19 91.08,37.19 92.71,35.56 JP2.13
PCC_D6  (via drill 0.45)
  Top 0.178: U$1.92 43.66,33.05 v45.21,31.5
  Bottom 0.254: JP2.12 96.16,38.1 94.94,36.88 92.13,36.88 91.37,37.64 75,37.64 73.08,39.55 44.63,39.55 43.69,38.61 43.69,33.02 v45.21,31.5
PCC_D7  (via drill 0.45)
  Top 0.178: U$1.93 43.26,39.58
  Top 0.254: v43.31,39.62 43.26,39.58
  Bottom 0.254: JP2.11 75.18,38.1 73.15,40.13 43.69,40.13 43.31,39.75 v43.31,39.62
PCC_D8  (via drill 0.45)
  Top 0.178: U$1.43 59.35,25.74
  Top 0.254: 59.35,25.74 65.53,19.56 68.52,19.56 v68.81,19.84
  Bottom 0.254: v68.81,19.84 88.42,19.84 92.76,24.18 94.56,24.18 95.2,24.82 95.2,26.62 JP2.20
PCC_D9  (via drill 0.45)
  Top 0.178: U$1.44 59.71,26.14
  Top 0.254: 59.71,26.14 65.79,20.07 67.31,20.07 v67.82,20.57
  Bottom 0.254: v67.82,20.57 68.47,20.57 68.49,20.6 69.12,20.6 69.14,20.57 86.61,20.57 JP2.19
PCC_D10  (via drill 0.45)
  Top 0.178: U$1.56 60.5,30.94
  Top 0.254: 60.5,30.94 v60.71,30.73 | JP2.22 97.79,24.13 97.79,21.59 92.46,21.59 88.39,25.65 v88.39,28.45
  Bottom 0.254: v60.71,30.73 62.28,29.16 67.18,29.16 67.64,28.7 88.14,28.7 v88.39,28.45
PCC_D11
  Top 0.178: U$1.57 58.01,31.34
  Top 0.254: 58.01,31.34 59.94,33.27 59.94,43.82 62.58,46.46 84.1,46.46 92.2,38.35 92.2,27.18 JP2.21
PCC_D12  (via drill 0.45)
  Top 0.178: U$1.58 50.79,31.74
  Top 0.254: 50.79,31.74 v50.55,31.5 | JP2.24 96.52,22.88 95.19,24.21 93.4,24.21 90.68,26.92 v90.68,31.24
  Bottom 0.254: v50.55,31.5 54.54,31.5 54.74,31.7 88.19,31.7 88.65,31.24 v90.68,31.24
PCC_D13  (via drill 0.45)
  Top 0.178: U$1.59 51.93,32.14
  Top 0.254: 51.93,32.14 v51.56,32.51 | v89.41,32 89.41,25.65 92.2,22.86 JP2.23
  Bottom 0.254: v51.56,32.51 52.12,31.95 54.35,31.95 54.55,32.16 89.26,32.16 v89.41,32
PCC_DEN1
  Top 0.178: U$1.60 58.45,32.54
  Top 0.254: 58.45,32.54 59.44,33.53 59.44,43.92 62.41,46.89 85.93,46.89 89.89,42.93 93.73,42.93 JP2.7
PCC_DEN2
  Top 0.178: U$1.61 58.09,32.94
  Top 0.254: 58.09,32.94 58.93,33.78 58.93,44.06 62.19,47.32 86.11,47.32 90,43.43 92.31,43.43 93.27,44.4 95.17,44.4 96.39,43.18 JP2.8
PCC_XCLK  (via drill 0.5)
  Top 0.178: U$1.85 46.46,43.46 44.85,45.06 v44.85,45.49
  Top 0.254: v91.61,44.44 91,45.06 89.59,45.06 86.47,48.18 75.51,48.18 v75.18,48.51
  Bottom 0.254: v44.85,45.49 47.02,43.32 50.8,43.32 52.07,44.59 70.02,44.59 70.7,45.27 72.45,45.27 75.18,48.01 v75.18,48.51 | JP2.10 96.17,40.64 94.96,41.86 93.54,41.86 92.53,42.87 92.53,43.52 v91.61,44.44
PWR_SWITCH
  Top 0.406: SW1.B 20.95,6.69 18.58,6.69 18.24,6.35 16.76,6.35 15.49,7.62 15.49,8.74 | JP1.1 15.49,11.9 R7.1
  Top 0.508: T2.3 15.49,8.74 JP1.1
PWRIN
  Top 1.016: X5.PWR 12.88,10.33 D1.A
RXLED  (via drill 0.5)
  Top 0.203: U$1.124 40.64,23.36 38.14,23.36 37.95,23.17 36.31,23.17 33.72,20.57 33.51,20.57 v33.02,20.09
  Top 0.254: v29.21,34.55 28.96,34.8 17.91,34.8 v17.4,34.29 | v16.76,28.19 13.72,28.19 13.23,28.68 R2.7
  Bottom 0.203: v33.02,20.09 33.35,20.42 33.35,20.83
  Bottom 0.254: 33.35,20.83 33.35,27.34 33.05,27.64 33.05,28.32 29.21,32.15 v29.21,34.55 | v17.4,34.29 17.4,28.7 16.76,28.07 v16.76,28.19
SCK  (via drill 0.45)
  Top 0.178: 62.68,27.74 U$1.48 44.4,27.74
  Top 0.254: v43.94,27.94 44.2,27.94 44.4,27.74 | 62.68,27.74 62.88,27.94 ICSP.3
  Bottom 0.254: JP2.33 53.09,10.16 51.77,11.48 51.77,23.22 50.86,24.13 47.76,24.13 v43.94,27.94
SCL  (via drill 0.45)
  Top 0.178: U$1.87 45.66,41.97
  Top 0.254: 45.66,41.97 44.96,42.67 v44.45,42.67 44.45,43.32 44.42,43.35 44.42,43.97 40.01,48.39 21.21,48.39 IOH.1
  Bottom 0.254: UART.8 78.28,42.72 70.93,42.72 70.03,43.62 52.39,43.62 50.48,41.71 45.72,41.71 44.76,42.67 v44.45,42.67
SCL_1  (via drill 0.45)
  Top 0.178: U$1.71 52.06,42.13
  Top 0.254: 52.06,42.13 v52.66,42.73
  Bottom 0.254: JP2.5 89.9,45.72 86.45,42.27 70.74,42.27 69.84,43.16 53.09,43.16 v52.66,42.73
SD_CD  (via drill 0.5)
  Top 0.203: v27.43,21.5 27.59,21.34 33.4,21.34 35.99,23.93 37.63,23.93 37.82,24.12 40.64,24.12 U$1.122
  Top 0.254: X1.CD1 17.94,25.18 18.41,25.65 21.84,25.65 v22.1,25.4
  Bottom 0.203: v22.1,25.4 22.25,25.24 22.25,23.19 23.95,21.5 v27.43,21.5
SD_CS  (via drill 0.5)
  Top 0.178: 32.36,31.34 U$1.104
  Top 0.203: 32.28,31.27 32.36,31.34
  Top 0.254: v25.86,23.16 25.86,22.97 24.61,21.71 9.78,21.71 7.34,19.28 X1.2 | v26.61,30.94 26.94,31.27 32.28,31.27
  Bottom 0.254: v25.86,23.16 25.86,23.62 25.96,23.71 25.96,30.29 v26.61,30.94
SD_MISO  (via drill 0.5)
  Top 0.178: U$1.105 33.73,30.94
  Top 0.254: 33.73,30.94 32.57,30.94 32.46,30.83 27.58,30.83 26.93,30.18 25.19,30.18 v24.13,31.24 | v22.99,23.5 22.5,23.01 11.15,23.01 9.27,24.89 6.49,24.89 X1.7
  Bottom 0.254: v24.13,31.24 24.13,24.64 v22.99,23.5
SD_MOSI  (via drill 0.5)
  Top 0.178: 29.43,32.14 U$1.102
  Top 0.203: 29.3,32.27 29.43,32.14
  Top 0.254: X1.3 6.92,20.38 8.68,22.15 24.18,22.15 24.96,22.93 24.96,23.78 v25.14,23.96 | v24.97,33.22 25.92,32.27 29.3,32.27
  Bottom 0.254: v25.14,23.96 25.53,24.35 25.53,32.66 v24.97,33.22
SD_SCK  (via drill 0.5)
  Top 0.203: U$1.103 24.91,31.74
  Top 0.254: X1.5 23.15,22.58 v24.07,23.5 | 24.91,31.74 v24.32,32.33
  Bottom 0.254: v24.07,23.5 24.07,23.97 25.02,24.91 25.02,31.64 v24.32,32.33
SDA  (via drill 0.45)
  Top 0.178: U$1.86 46.06,42.59
  Top 0.254: 46.06,42.59 45.18,43.46 v45.18,43.66 45.18,44.09 40.37,48.9 23.24,48.9 IOH.2
  Bottom 0.254: UART.7 83.82,49.02 77.98,43.18 71.12,43.18 70.23,44.07 52.2,44.07 50.29,42.16 45.97,42.16 45.18,42.95 v45.18,43.66
SDA_1  (via drill 0.45)  (1 unrouted)
  Top 0.178: U$1.70 52.46,40.78
  Top 0.254: 52.46,40.78 v53.59,41.91
  Bottom 0.254: 96.77,45.59 95.56,44.37 93.53,44.37 92.64,45.26 90.09,45.26 86.64,41.81 70.55,41.81 69.77,42.59 54.27,42.59 v53.59,41.91
SS  (via drill 0.45)
  Top 0.178: U$1.49 45.27,28.14
  Top 0.254: 45.27,28.14 44.96,28.45 v44.96,28.96
  Bottom 0.254: JP2.34 95.3,11.38 92.51,11.38 91.75,10.62 53.27,10.62 52.22,11.67 52.22,23.41 51.05,24.58 47.95,24.58 44.96,27.57 v44.96,28.96
SWCLK  (via drill 0.45)
  Top 0.178: U$1.119 42.1,25.34 v42.93,26.16
  Top 0.254: X2.4 79.25,13.59 78.49,12.83 78.49,11.68 81.28,8.89 85.6,8.89 86.36,8.13 v86.61,8.13 87.38,8.89 R4.1
  Bottom 0.254: v42.93,26.16 39.88,23.11 39.88,11.43 42.42,8.89 61.72,8.89 64.97,5.64 66.86,5.64 70.16,8.94 85.8,8.94 v86.61,8.13
SWDIO  (via drill 0.45)
  Top 0.178: U$1.120 42.88,24.94
  Top 0.254: 42.88,24.94 v42.93,24.89 | X2.2 80.27,10.91 81.79,9.4 v86.61,9.4
  Bottom 0.254: v86.61,9.4 67.06,9.4 66.86,9.6 65.22,9.6 65.02,9.4 42.93,9.4 42.42,9.91 42.42,24.38 v42.93,24.89
SWO  (via drill 0.45)
  Top 0.178: U$1.121 37.44,24.54
  Top 0.254: 37.44,24.54 v37.34,24.64 | X2.6 79.25,14.86 77.98,13.59 77.98,11.44 81.03,8.38 84.71,8.38 86.08,7.01 v86.77,7.01
  Bottom 0.254: v37.34,24.64 39.12,22.86 39.12,11.54 42.23,8.43 61.53,8.43 64.78,5.18 67.05,5.18 70.35,8.48 85.19,8.48 86.66,7.01 v86.77,7.01
TXLED  (via drill 0.5)
  Top 0.203: U$1.123 37.98,23.74 37.79,23.55 36.15,23.55 33.56,20.95 32.64,20.95 32.29,20.6 v32,20.6
  Top 0.254: v28.45,36.78 26.9,35.23 17.14,35.23 16.64,34.73 v16.64,33.52 | v15.99,27.44 15.74,27.69 13.46,27.69 12.43,28.72 R2.6
  Bottom 0.203: v32,20.6 32.92,21.52 32.92,21.76
  Bottom 0.254: 32.92,21.76 32.92,27.16 32.62,27.46 32.62,28.14 28.46,32.3 28.46,36.77 v28.45,36.78 | v16.64,33.52 16.89,33.27 16.89,29.52 15.99,28.62 v15.99,27.44
UART1_RX  (via drill 0.45)
  Top 0.178: U$1.42 58.99,25.34
  Top 0.254: 58.99,25.34 65.28,19.05 69.09,19.05 69.85,19.81 69.85,41.91 71.88,43.94 v72.39,43.94
  Bottom 0.254: UART.6 81.28,47.24 77.98,43.94 v72.39,43.94
UART1_TX  (via drill 0.45)
  Top 0.178: U$1.41 58.63,24.94
  Top 0.254: 58.63,24.94 65.08,18.49 69.29,18.49 70.36,19.56 70.36,41.66 71.91,43.21 72.69,43.21 73.12,43.64 73.12,44.42 v73.41,44.7
  Bottom 0.254: UART.5 78.74,45.97 77.47,44.7 v73.41,44.7
UART2_RX  (via drill 0.45)
  Top 0.178: U$1.77 49.66,43.81
  Top 0.254: 49.66,43.81 v49.28,44.2
  Bottom 0.254: UART.4 71.58,46.18 50.29,46.18 49.28,45.16 v49.28,44.2
UART2_TX  (via drill 0.45)
  Top 0.178: U$1.76 50.06,44.68
  Top 0.254: v49.22,46.23 49.22,45.52 50.06,44.68
  Bottom 0.254: UART.3 69.49,46.63 49.78,46.63 49.38,46.23 v49.22,46.23
UART3_RX  (via drill 0.45)
  Top 0.178: U$1.83 47.26,45.07
  Top 0.203: 47.26,45.07 46.61,45.72
  Top 0.254: v46.48,45.72 46.61,45.72
  Bottom 0.254: UART.2 67.41,47.09 46.74,47.09 46.48,46.84 v46.48,45.72
UART3_TX  (via drill 0.45)
  Top 0.203: 47.66,45.92 U$1.82
  Top 0.254: v45.21,46.99 46.59,46.99 47.66,45.92
  Bottom 0.254: UART.1 68.58,50.05 66.08,47.55 46.28,47.55 45.72,46.99 v45.21,46.99
USB_HOSTEN  (via drill 0.5)
  Top 0.178: 34.29,28.7 35.25,27.74 U$1.113
  Top 0.254: 34.29,28.7 33.02,28.7 31.98,27.66 v30.73,27.66 | R11.2 23.37,31.91 23.37,30.8 24.84,29.34 v29.21,29.34
  Bottom 0.254: v30.73,27.66 29.21,29.18 v29.21,29.34
USBVCC
  Top 0.61: F2.2 10.82,33.36 9.86,32.4 9.86,26.34 12.45,23.75 19.38,23.75 TR1.1
USHIELD
  Top 0.229: 2.72,41.4 2.72,39.25 X3.BASE@1 X3.BASE@2
  Top 0.254: FB2.2 2.42,43.88 X3.SPRT@3
  Top 0.406: X3.SPRT@2 4.92,34.5 X3.SPRT@4 | X3.SPRT@3 2.72,41.4 X3.SPRT@1
  pour Bottom (rank 3): 0.13,43.05 0.13,32.89 6.35,32.89 6.35,43.05
  pour Top (rank 2): 0.13,43.05 0.13,32.89 6.35,32.89 6.35,43.05
VBUS  (via drill 0.5)
  Top 0.406: X3.VBUS 6.89,39.4 v7.75,40.26
  Top 0.61: v7.75,35.69 7.98,35.46 F2.1
  Bottom 0.61: v7.75,40.26 v7.75,35.69
VDDCORE
  Top 0.178: U$1.115 29.39,26.94
  Top 0.254: C8.2 30.82,24.75 L1.P$1 30.71,24.93 C1.1 29.09,27.04 C9.1 29.39,26.94
VIN
  Top 0.254: R1.1 25.49,24.68 26.62,23.55 26.62,22.84 24.37,20.59 24.37,19.3 24.78,19.3 PC1.+
  Top 0.61: 21.34,8.38 18.14,8.38 T2.1 | 21.34,8.38 21.34,13.21 22.64,14.52 U1.3 | POWER.8 45.72,4.83 45.09,5.46 35.56,5.46 34.79,6.22 27.05,6.22 24.89,8.38 21.34,8.38
  Top 1.27: U1.3 24.37,14.71 24.37,19.3 C12.1

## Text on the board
tNames: 1 | 1 | DIGITAL
214bmp: D:/SmartProjects/Snc/a4_bn_logo2.bmp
